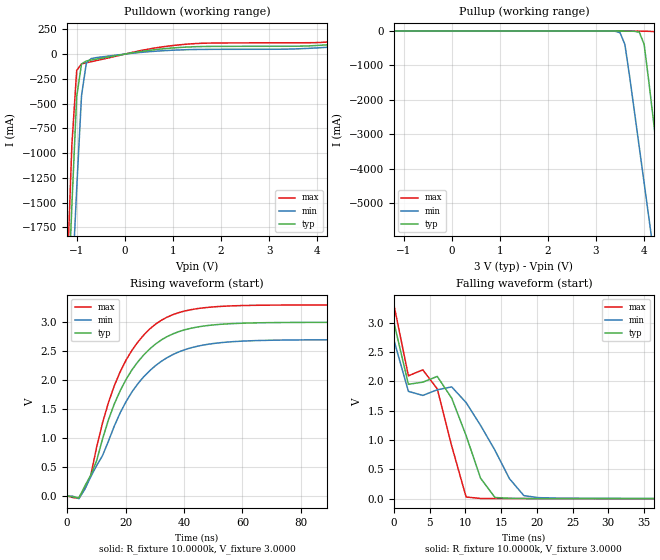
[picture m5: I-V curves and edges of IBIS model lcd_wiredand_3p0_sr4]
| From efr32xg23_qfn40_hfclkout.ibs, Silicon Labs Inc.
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|   Model lcd_wiredand_3p0_sr4
[Model]  lcd_wiredand_3p0_sr4
Model_type Output
Polarity   Inverting
Enable   Active-Low
C_comp   1.6300pF   1.4000pF   2.7000pF
[Temperature Range]   25.0000   0.1250k   -40.0000
[Pullup Reference]   3.0000V   2.7000V   3.3000V
[Pulldown Reference]   0.0V   0.0V   0.0V
[POWER Clamp Reference]   3.0000V   2.7000V   3.3000V
[GND Clamp Reference]   0.0V   0.0V   0.0V
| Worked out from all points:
|   slope of the pulldown table from 0 to 0.45 V, typ, clamps not added: 13.2 ohm
|   rising waveform, R_fixture 10.0000k, V_fixture 3.0000: 20-80 % time 15.6ns typ, 17.9ns min, 14.6ns max; typ from 0.003 V to 3 V
|   falling waveform, R_fixture 10.0000k, V_fixture 3.0000: 20-80 % time 10.3ns typ, 14.1ns min, 7.53ns max; typ from 3 V to 0.003 V
[Pulldown]
|Voltage   I(typ)   I(min)   I(max)
-3V       -24.3A     -21.99A    -26.6A
-1.2V     -2.716A    -3.412A    -2.254A
-1.1V     -1.526A    -2.385A    -915.6mA
-1V       -429.7mA   -1.36A     -165.3mA
-900mV    -99.37mA   -421mA     -98.78mA
-800mV    -69.26mA   -90.62mA   -87.32mA
-700mV    -59.97mA   -45.41mA   -76.82mA
400mV     30.95mA    19.99mA    42.35mA
1.1V      65.5mA     41.43mA    91.79mA
4.2V      93.5mA     68.54mA    121.5mA
5.1V      135.6mA    103.8mA    168.6mA
6V        196.8mA    153.8mA    241.9mA
[Pullup]
|Voltage   I(typ)   I(min)   I(max)
-3V       338.2nA    9.289uA    587.2nA
3.5V      -430.7uA   -50.4mA    -8.469nA
3.6V      -1.559mA   -390.7mA   -692.6nA
4V        -385.8mA   -4.417A    -4.219mA
4.1V      -1.495A    -5.446A    -8.403mA
4.2V      -2.686A    -6.476A    -14.95mA
4.3V      -3.882A    -7.507A    -84.19mA
4.4V      -5.077A    -8.538A    -881.8mA
4.5V      -6.274A    -9.569A    -2.22A
4.7V      -8.669A    -11.63A    -4.917A
4.8V      -9.867A    -12.66A    -6.266A
6V        -24.27A    -25.05A    -22.51A
[Ramp]
| variable   typ   min   max
dV/dt_r  -0.1715m/17.0894p   -0.1952m/53.1666p   -0.1328m/7.7808p
dV/dt_f  1.7980/10.2704n   1.6171/14.0753n   1.9783/7.5313n
R_load = 10.0000k
[Rising Waveform]
R_fixture= 10.0000k
V_fixture= 3.0000
V_fixture_min= 2.7000
V_fixture_max= 3.3000
|time   V(typ)   V(min)   V(max)
0s        3.394mV    4.689mV    2.757mV
4.04ns    -27.8mV    -43.18mV   -33.37mV
8.081ns   360.8mV    333.8mV    353.5mV
14.14ns   1.315V     948.1mV    1.614V
18.18ns   1.821V     1.44V      2.147V
22.22ns   2.181V     1.801V     2.519V
30.3ns    2.627V     2.254V     2.97V
38.38ns   2.842V     2.493V     3.17V
66.67ns   2.992V     2.687V     3.295V
200ns     3V         2.7V       3.3V
[Falling Waveform]
R_fixture= 10.0000k
V_fixture= 3.0000
V_fixture_min= 2.7000
V_fixture_max= 3.3000
|time   V(typ)   V(min)   V(max)
0s        3V         2.7V       3.3V
2.02ns    1.949V     1.829V     2.094V
4.04ns    1.986V     1.76V      2.195V
6.061ns   2.084V     1.856V     1.871V
10.1ns    1.077V     1.638V     31.55mV
12.12ns   352.3mV    1.251V     6.885mV
14.14ns   22.67mV    826.3mV    4.835mV
18.18ns   7.004mV    55.1mV     3.689mV
20.2ns    5.818mV    20.84mV    3.454mV
200ns     3.395mV    4.693mV    2.758mV
